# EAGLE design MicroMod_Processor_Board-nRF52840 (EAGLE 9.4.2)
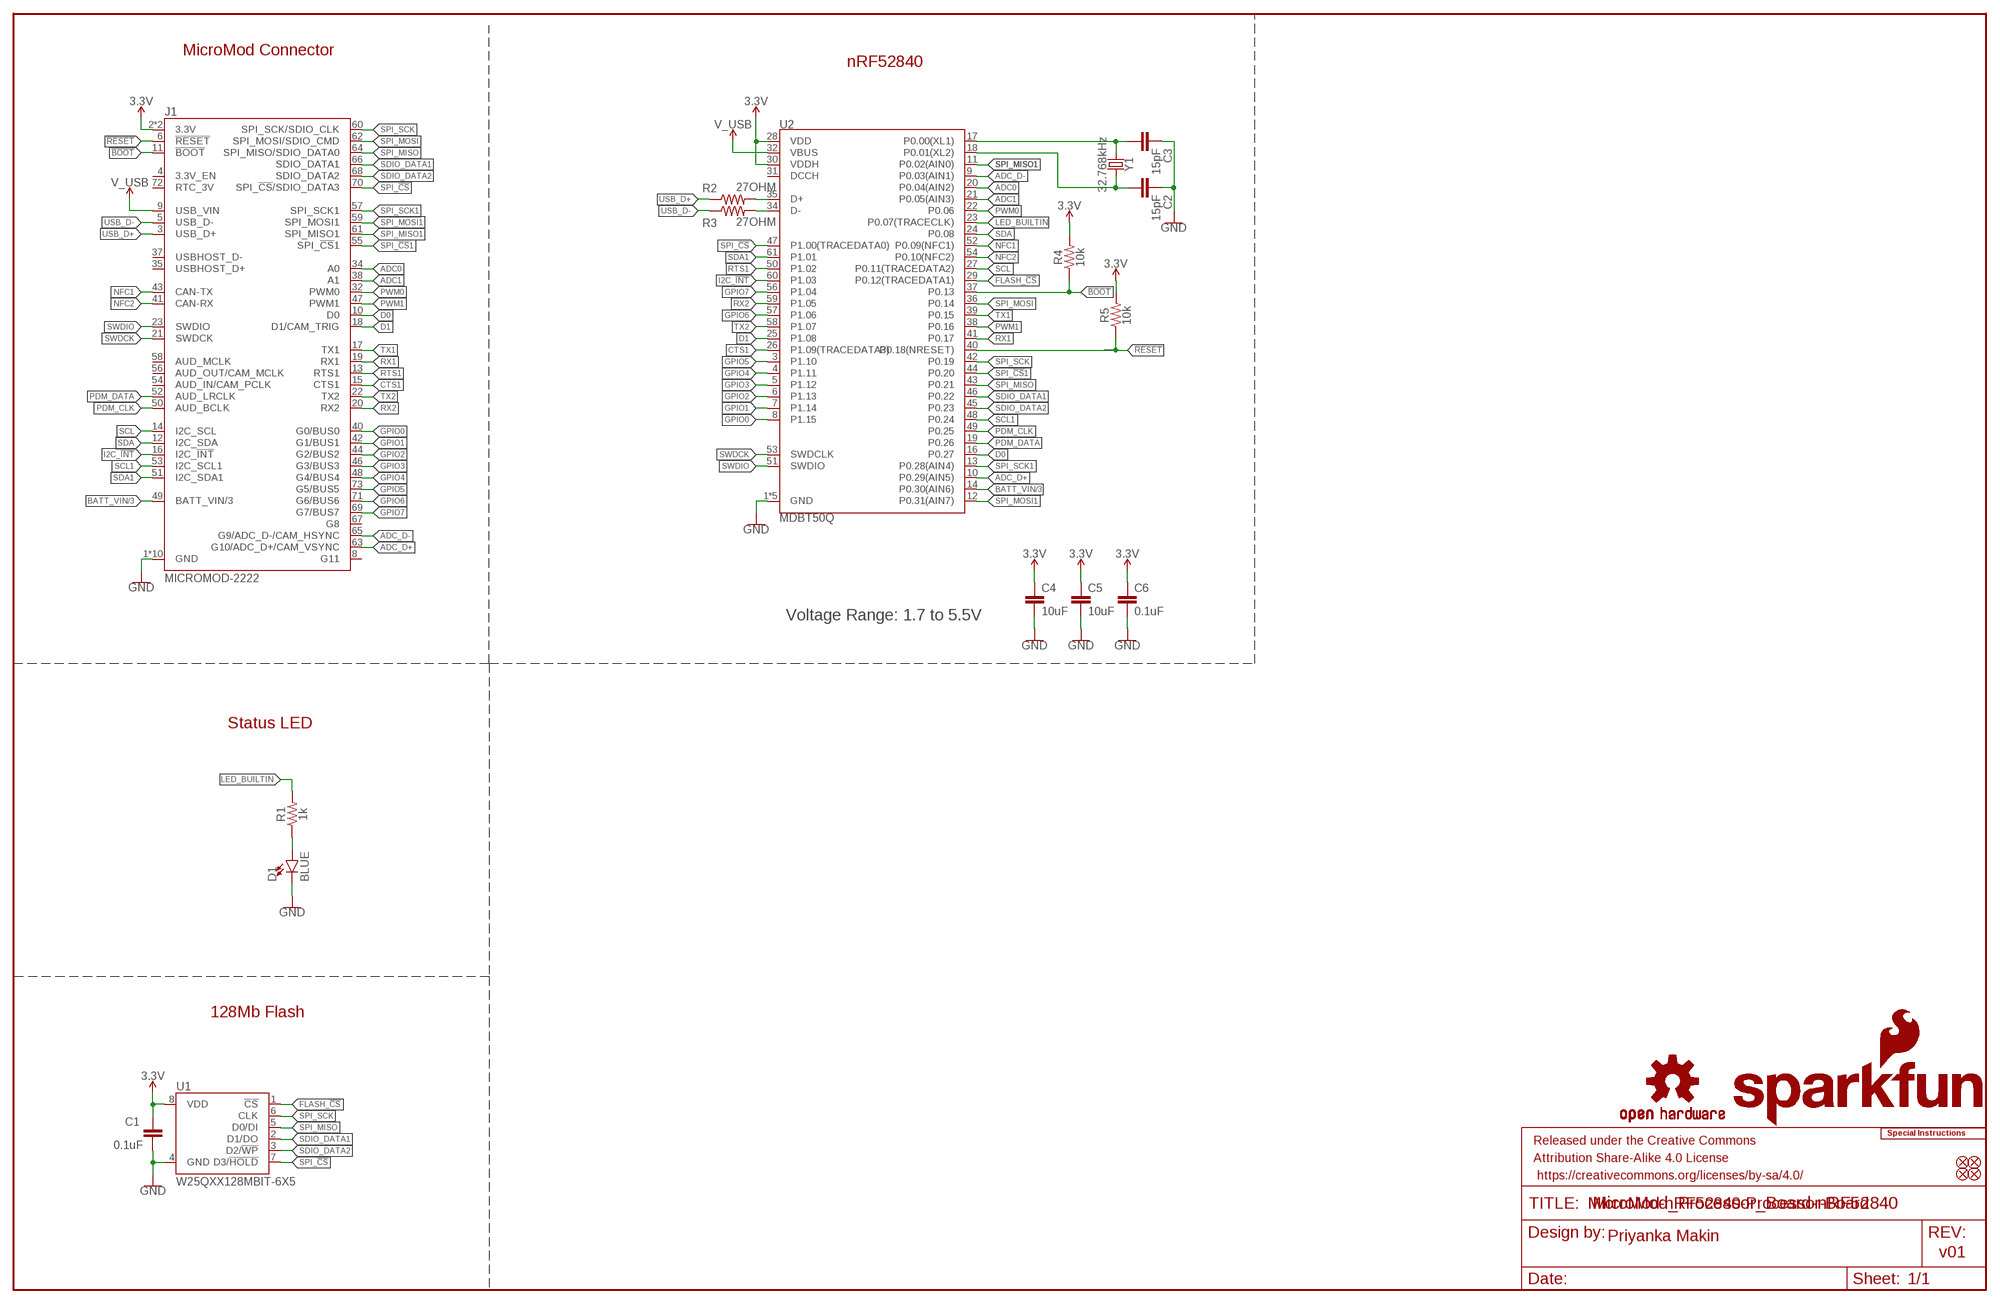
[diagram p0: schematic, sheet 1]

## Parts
C1  0.1uF  0.1UF-0402T-16V-10%  [0402-TIGHT]
C2  15pF  15PF-0402T-50V-5%  [0402-TIGHT]
C3  15pF  15PF-0402T-50V-5%  [0402-TIGHT]
C4  10uF  10UF-0402T-6.3V-20%  [0402-TIGHT]
C5  10uF  10UF-0402T-6.3V-20%  [0402-TIGHT]
C6  0.1uF  0.1UF-0402T-16V-10%  [0402-TIGHT]
D1  BLUE  LED-BLUE0603  [LED-0603]
FD1  FIDUCIALUFIDUCIAL  [FIDUCIAL-MICRO]
FD2  FIDUCIALUFIDUCIAL  [FIDUCIAL-MICRO]
FD3  FIDUCIALUFIDUCIAL  [FIDUCIAL-MICRO]
FD4  FIDUCIALUFIDUCIAL  [FIDUCIAL-MICRO]
FRAME1  FRAME-LEDGER  [CREATIVE_COMMONS]
J1  MICROMOD-2222  [M.2-CARD-E-22]
LOGO1  SFE_LOGO_NAME_FLAME.1_INCH  [SFE_LOGO_NAME_FLAME_.1]
LOGO2  SFE_LOGO_FLAME.1_INCH  [SFE_LOGO_FLAME_.1]
LOGO3  OSHW-LOGOMINI  [OSHW-LOGO-MINI]
LOGO4  SPECIAL_INSTRUCTIONS-ORDERING  [ORDERING_INSTRUCTIONS]
R1  1k  1KOHM-0402T-1/16W-1%  [0402-TIGHT]
R2  27OHM  [0402-TIGHT]
R3  27OHM  [0402-TIGHT]
R4  10k  10KOHM-0402T-1/16W-1%  [0402-TIGHT]
R5  10k  10KOHM-0402T-1/16W-1%  [0402-TIGHT]
U1  W25QXX128MBIT-6X5  [WSON-8-6X5]
U2  MDBT50Q  [MDBT50Q]
Y1  32.768kHz  CRYSTAL-32.768KHZSMD-3.2X1.5  [CRYSTAL-SMD-3.2X1.5MM]

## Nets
3.3V: C1.1 C4.1 C5.1 C6.1 J1.2(3.3V) J1.74(3.3V) R4.2 R5.2 U1.8(VDD) U2.28(VDD) U2.30(VDDH)
!BOOT!: J1.11(!BOOT!) R4.1 U2.37(P0.13)
!RESET!: J1.6(!RESET!) R5.1 U2.40(P0.18(NRESET))
ADC0: J1.34(A0) U2.20(P0.04(AIN2))
ADC1: J1.38(A1) U2.21(P0.05(AIN3))
ADC_D+: J1.63(G10/ADC_D+/CAM_VSYNC) U2.10(P0.29(AIN5))
ADC_D-: J1.65(G9/ADC_D-/CAM_HSYNC) U2.9(P0.03(AIN1))
BATT_VIN/3: J1.49(BATT_VIN/3) U2.14(P0.30(AIN6))
CTS1: J1.15(CTS1) U2.26(P1.09(TRACEDATA3))
D0: J1.10(D0) U2.16(P0.27)
D1: J1.18(D1/CAM_TRIG) U2.25(P1.08)
FLASH_!CS!: U1.1(!CS!) U2.29(P0.12(TRACEDATA1))
GND: C1.2 C2.1 C3.1 C4.2 C5.2 C6.2 D1.C J1.1(GND) J1.7(GND) J1.33(GND) J1.36(GND) J1.39(GND) J1.45(GND) J1.75(GND) J1.GND1(GND) J1.GND2(GND) J1.GND3(GND) U1.4(GND) U2.1(GND) U2.2(GND) U2.15(GND) U2.33(GND) U2.55(GND)
GPIO0: J1.40(G0/BUS0) U2.8(P1.15)
GPIO1: J1.42(G1/BUS1) U2.7(P1.14)
GPIO2: J1.44(G2/BUS2) U2.6(P1.13)
GPIO3: J1.46(G3/BUS3) U2.5(P1.12)
GPIO4: J1.48(G4/BUS4) U2.4(P1.11)
GPIO5: J1.73(G5/BUS5) U2.3(P1.10)
GPIO6: J1.71(G6/BUS6) U2.57(P1.06)
GPIO7: J1.69(G7/BUS7) U2.56(P1.04)
I2C_!INT!: J1.16(I2C_!INT!) U2.60(P1.03)
LED_BUILTIN: R1.2 U2.23(P0.07(TRACECLK))
N$1: R2.2 U2.35(D+)
N$2: D1.A R1.1
N$3: R3.2 U2.34(D-)
N$4: C3.2 U2.17(P0.00(XL1)) Y1.P$1
N$6: C2.2 U2.18(P0.01(XL2)) Y1.P$2
NFC1: J1.43(CAN-TX) U2.52(P0.09(NFC1))
NFC2: J1.41(CAN-RX) U2.54(P0.10(NFC2))
PDM_CLK: J1.50(AUD_BCLK) U2.49(P0.25)
PDM_DATA: J1.52(AUD_LRCLK) U2.19(P0.26)
PWM0: J1.32(PWM0) U2.22(P0.06)
PWM1: J1.47(PWM1) U2.38(P0.16)
RTS1: J1.13(RTS1) U2.50(P1.02)
RX1: J1.19(RX1) U2.41(P0.17)
RX2: J1.20(RX2) U2.59(P1.05)
SCL: J1.14(I2C_SCL) U2.27(P0.11(TRACEDATA2))
SCL1: J1.53(I2C_SCL1) U2.48(P0.24)
SDA: J1.12(I2C_SDA) U2.24(P0.08)
SDA1: J1.51(I2C_SDA1) U2.61(P1.01)
SDIO_DATA1: J1.66(SDIO_DATA1) U1.2(D1/DO) U2.46(P0.22)
SDIO_DATA2: J1.68(SDIO_DATA2) U1.3(D2/!WP!) U2.45(P0.23)
SPI_!CS!: J1.70(SPI_!CS!/SDIO_DATA3) U1.7(D3/!HOLD!) U2.47(P1.00(TRACEDATA0))
SPI_!CS!1: J1.55(SPI_!CS!1) U2.44(P0.20)
SPI_MISO: J1.64(SPI_MISO/SDIO_DATA0) U1.5(D0/DI) U2.43(P0.21)
SPI_MISO1: J1.61(SPI_MISO1) U2.11(P0.02(AIN0))
SPI_MOSI: J1.62(SPI_MOSI/SDIO_CMD) U2.36(P0.14)
SPI_MOSI1: J1.59(SPI_MOSI1) U2.12(P0.31(AIN7))
SPI_SCK: J1.60(SPI_SCK/SDIO_CLK) U1.6(CLK) U2.42(P0.19)
SPI_SCK1: J1.57(SPI_SCK1) U2.13(P0.28(AIN4))
SWDCK: J1.21(SWDCK) U2.53(SWDCLK)
SWDIO: J1.23(SWDIO) U2.51(SWDIO)
TX1: J1.17(TX1) U2.39(P0.15)
TX2: J1.22(TX2) U2.58(P1.07)
USB_D+: J1.3(USB_D+) R2.1
USB_D-: J1.5(USB_D-) R3.1
V_USB: J1.9(USB_VIN) U2.32(VBUS)
Unconnected: J1.4(3.3V_EN) J1.8(G11) J1.35(USBHOST_D+) J1.37(USBHOST_D-) J1.54(AUD_IN/CAM_PCLK) J1.56(AUD_OUT/CAM_MCLK) J1.58(AUD_MCLK) J1.67(G8) J1.72(RTC_3V) U2.31(DCCH)

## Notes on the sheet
- MicroMod Connector
- nRF52840
- Voltage Range: 1.7 to 5.5V
- Status LED
- 128Mb Flash
- MicroMod-nRF52840-Processor-Board
- Priyanka Makin
- v01

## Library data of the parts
C1 C6 = SparkFun-Capacitors:0.1UF: 0.1µF ceramic capacitors; PROD_ID: CAP-12416
C2 C3 = SparkFun-Capacitors:15PF: 15pF ceramic capacitors; PROD_ID: CAP-13063
C4 C5 = SparkFun-Capacitors:10UF: 10.0µF ceramic capacitors; PROD_ID: CAP-14848
D1 = SparkFun-LED:LED-BLUE: Blue SMD LED; PROD_ID: DIO-08575
FD1-FD4 = SparkFun-Aesthetics:FIDUCIAL: Fiducial Alignment Points
FRAME1 = SparkFun-Aesthetics:FRAME-LEDGER: Schematic Frame - Ledger
J1 = SparkFun-MicroMod:MICROMOD: MicroMod Connector Description: A card edge connector and mating PCB connector to allow various MicroMod Processor Boards to be coupled with various carrier boards of different capabilities. Based on the M.2 standard.
LOGO1 = SparkFun-Aesthetics:SFE_LOGO_NAME_FLAME: SparkFun Font Logo w/ Flame
LOGO2 = SparkFun-Aesthetics:SFE_LOGO_FLAME: SparkFun Flame Logo
LOGO3 = SparkFun-Aesthetics:OSHW-LOGO: Open-Source Hardware (OSHW) Logo
LOGO4 = SparkFun-Aesthetics:SPECIAL_INSTRUCTIONS: Special Ordering/Production Instructions Alert
R1 = SparkFun-Resistors:1KOHM: 1kΩ resistor; PROD_ID: RES-14342
R2 R3 = SparkFun-Resistors:27OHM: 27Ω resistor
R4 R5 = SparkFun-Resistors:10KOHM: 10kΩ resistor; PROD_ID: RES-14241
U1 = SparkFun-MicroMod:W25QXX; PROD_ID: IC-15107
U2 = SparkFun-RF:MDBT50Q; PROD_ID: IC-14109
Y1 = SparkFun-Clocks:CRYSTAL-32.768KHZ: 32.768kHz Crystal; PROD_ID: XTAL-13062

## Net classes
0 default: width 0 mm, drill 0 mm

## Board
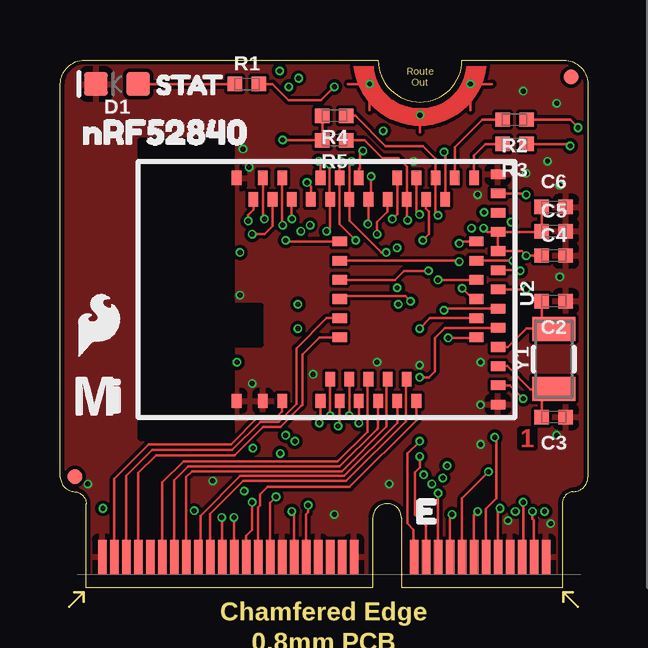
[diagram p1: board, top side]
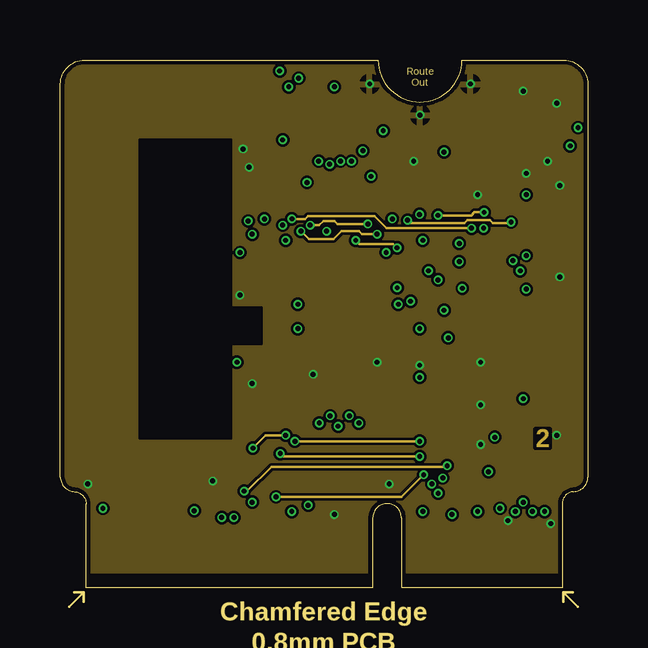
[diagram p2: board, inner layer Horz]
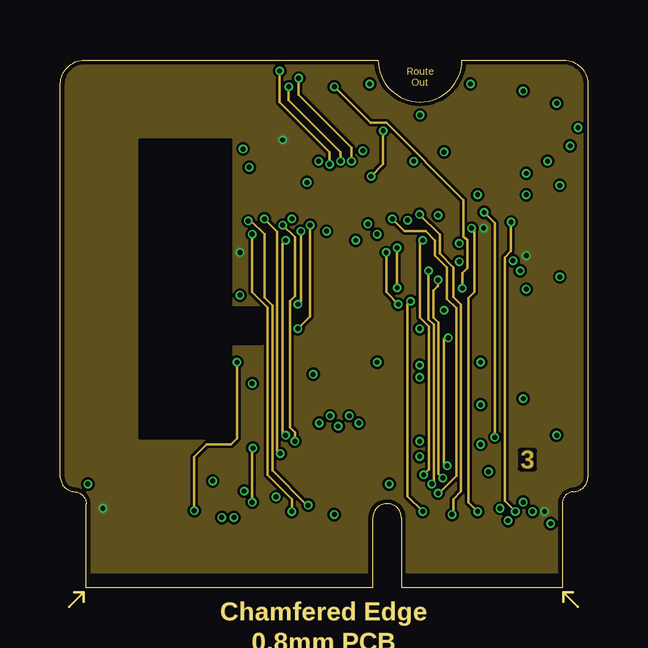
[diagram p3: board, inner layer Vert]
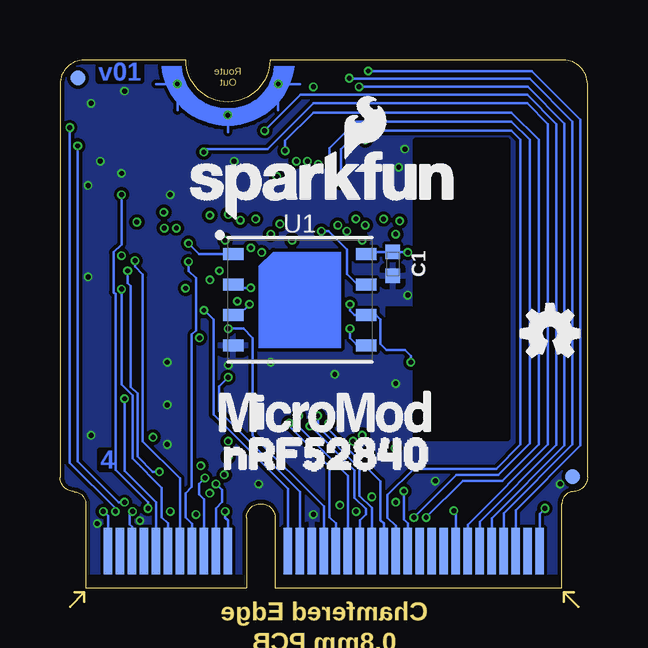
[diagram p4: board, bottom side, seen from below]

Size 22 x 22 mm. Coordinates in mm from the lower left corner, seen from the top.
Outline: 0,4.6 0,21 arc-87 1,22 13.25,22 arc180 16.75,22 21,22 arc-87 22,21 22,4.6
Outline: 0,4.6 arc87 0.6,4
Outline: 21.4,4 arc87 22,4.6
Outline: 21.4,4 arc85 20.93,3.5 20.93,0 14.22,0 14.22,2.9 arc180 13.03,2.9 13.03,0 1.07,0 1.07,3.5 arc84 0.6,4
Outline: 21.4,4 arc87 22,4.6
Outline: 0,4.6 arc87 0.6,4
Copper layers (1+2*15+16): Top 0.035mm / dielectric 1.5mm / Horz 0.035mm / dielectric 0.15mm / Vert 0.035mm / dielectric 0.2mm / Bottom 0.035mm
Design rules "SparkFun-4-layer-MicroMod": minimum track width 4mil, minimum drill 0.2mm, track to track 4mil, track to pad 4mil, pad to pad 4mil, via to via 4mil, smd to smd 4mil, copper to edge 6mil, drill to drill 6mil, minimum pad ring 3mil, minimum via ring 3mil, stop-mask expansion 4mil, vias tented up to drill 25mil, thermal gap 10mil

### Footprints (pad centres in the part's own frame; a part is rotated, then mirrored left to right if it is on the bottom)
0402-TIGHT = smd 0.6 x 0.6: 1 -0.5,0; 2 0.5,0
LED-0603 = smd 1 x 1: A -0.877,0; C 0.877,0
FIDUCIAL-MICRO = smd 0.635 x 0.635: 1 0,0
M.2-CARD-E-22 = smd 0.35 x 1.45: 1 9.25,1.275; 3 8.75,1.275; 5 8.25,1.275; 7 7.75,1.275; 9 7.25,1.275; 11 6.75,1.275; 13 6.25,1.275; 15 5.75,1.275; 17 5.25,1.275; 19 4.75,1.275; 21 4.25,1.275; 23 3.75,1.275; 33 1.25,1.275; 35 0.75,1.275; 37 0.25,1.275; 39 -0.25,1.275; 41 -0.75,1.275; 43 -1.25,1.275; 45 -1.75,1.275; 47 -2.25,1.275; 49 -2.75,1.275; 51 -3.25,1.275; 53 -3.75,1.275; 55 -4.25,1.275; 57 -4.75,1.275; 59 -5.25,1.275; 61 -5.75,1.275; 63 -6.25,1.275; 65 -6.75,1.275; 67 -7.25,1.275; 69 -7.75,1.275; 71 -8.25,1.275; 73 -8.75,1.275; 75 -9.25,1.275 | smd 0.35 x 1.95 bottom: 2 9,1.525; 4 8.5,1.525; 6 8,1.525; 8 7.5,1.525; 10 7,1.525; 12 6.5,1.525; 14 6,1.525; 16 5.5,1.525; 18 5,1.525; 20 4.5,1.525; 22 4,1.525; 32 1.5,1.525; 34 1,1.525; 36 0.5,1.525; 38 0,1.525; 40 -0.5,1.525; 42 -1,1.525; 44 -1.5,1.525; 46 -2,1.525; 48 -2.5,1.525; 50 -3,1.525; 52 -3.5,1.525; 54 -4,1.525; 56 -4.5,1.525; 58 -5,1.525; 60 -5.5,1.525; 62 -6,1.525; 64 -6.5,1.525; 66 -7,1.525; 68 -7.5,1.525; 70 -8,1.525; 72 -8.5,1.525; 74 -9,1.525 | drill 0.2: GND1 1.9,21; GND2 4,19.7; GND3 6.1,21
WSON-8-6X5 = smd 0.85 x 0.5: 1 -2.775,1.905; 2 -2.775,0.635; 3 -2.775,-0.635; 4 -2.775,-1.905; 5 2.775,-1.905; 6 2.775,-0.635; 7 2.775,0.635; 8 2.775,1.905
MDBT50Q = smd 0.6 x 0.4: 1 -4.65,3.65; 2 -4.65,2.55; 3 -4.65,1.75; 4 -4.65,0.15; 5 -3.75,-0.25; 6 -4.65,-0.65; 7 -3.75,-1.05; 8 -4.65,-1.45; 9 -3.75,-1.85; 10 -4.65,-2.25; 11 -3.75,-2.65; 12 -4.65,-3.05; 13 -3.75,-3.45; 14 -4.65,-3.85; 34 4.65,-6.25; 35 4.65,-5.45; 36 3.75,-5.05; 37 4.65,-4.65; 38 3.75,-4.25; 39 4.65,-3.85; 40 3.75,-3.45; 41 4.65,-3.05; 42 3.75,-2.65; 43 3.75,-1.85; 44 4.65,-1.45; 45 3.75,-1.05; 46 4.65,-0.65; 47 3.75,-0.25; 48 4.65,0.15; 49 3.75,0.55; 50 3.75,1.35; 51 4.65,1.75; 52 3.75,2.15; 53 4.65,2.55; 54 3.75,2.95; 55 4.65,3.65 | smd 0.4 x 0.6: 15 -4.8,-7.25; 16 -4,-7.25; 17 -3.2,-7.25; 18 -2.4,-7.25; 19 -2,-6.35; 20 -1.6,-7.25; 21 -1.2,-6.35; 22 -0.8,-7.25; 23 -0.4,-6.35; 24 0,-7.25; 25 0.4,-6.35; 26 0.8,-7.25; 27 1.2,-6.35; 28 1.6,-7.25; 29 2,-6.35; 30 2.4,-7.25; 31 3.2,-7.25; 32 4,-7.25; 33 4.8,-7.25; 56 -2,-0.65; 57 -1.2,-0.65; 58 -0.4,-0.65; 59 0.4,-0.65; 60 1.2,-0.65; 61 2,-0.65
CRYSTAL-SMD-3.2X1.5MM = smd 1 x 1.8: P$1 -1.25,0; P$2 1.25,0

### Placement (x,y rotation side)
C1  8.12,13.49 270 bottom
C2  20.57,11.94 180 top
C3  20.57,7.11 180 top
C4  20.57,13.84 0 top
C5  20.57,14.86 0 top
C6  20.57,15.88 0 top
D1  2.37,21 180 top
FD1  0.62,4.62 0 top
FD2  21.3,21.3 0 top
FD3  21.25,21.25 0 bottom
FD4  0.62,4.62 0 bottom
FRAME1  not placed on the board
J1  11,0 0 top
LOGO1  11,16.79 0 bottom
LOGO2  1.6,10.95 0 top
LOGO3  1.56,10.61 0 bottom
LOGO4  not placed on the board
R1  7.78,21 0 top
R2  18.94,19.51 180 top
R3  18.94,18.49 180 top
R4  11.43,19.67 180 top
R5  11.43,18.65 180 top
U1  12,12 0 bottom
U2  11,12.43 90 top
U$1  [MICROMOD_MI_LOGO_.35]  1.55,8 0 top
U$2  [NRF528400]  16.36,5.58 0 bottom
U$3  [NRF528400]  0,19 0 top
U$4  [STAT_TO_32]  3.25,20.96 0 top
U$5  [MICROMOD_LOGO_.35]  11,7.3 0 bottom
Y1  20.57,9.53 90 top

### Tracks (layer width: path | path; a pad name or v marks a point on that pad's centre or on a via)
3.3V  (via drill 0.2)
  Top 0.102: U2.30 20.05,14.83 C5.1 C6.1 | C4.1 v19.43,13.84 19.24,14.03 U2.28 U2.30 | R4.2 R5.2 9.29,18.65 v9.27,18.67 | U2.30 17.81,14.83 v17.65,14.99
  Bottom 0.102: J1.2 20,2.98 v20.19,3.17 | J1.74 2,3.08 v1.78,3.3 | U1.8 9.14,13.99 C1.1 7.52,13.99 v7.49,13.97
  pour Vert (isolate 0.102): 0,22 22,22 22,0.64 0,0.64
  cutout Vert (isolate 0.305): 3.3,18.67 7.11,18.67 7.11,11.68 8.38,11.68 8.38,10.16 7.11,10.16 7.11,6.22 3.3,6.22
!BOOT!  (via drill 0.2)
  Top 0.102: R4.1 12.31,19.67 13.56,18.41 15.11,18.41 15.65,17.88 U2.37 15.65,15.62 v15.75,15.52 | v18.12,6.27 18.19,6.2 18.19,3.71 17.75,3.27 J1.11
  Horz 0.102: v15.75,15.52 17.14,15.52 17.27,15.65 v17.67,15.65
  Vert 0.102: v17.67,15.65 18.12,15.2 v18.12,6.27
!RESET!  (via drill 0.2)
  Top 0.102: R5.1 12.69,18.65 13.44,17.91 14.1,17.91 14.45,17.55 U2.40 14.45,15.34 v14.48,15.32
  Horz 0.102: v18.8,15.24 18.75,15.19 18.03,15.19 17.91,15.32 16.97,15.32 16.84,15.19 14.61,15.19 v14.48,15.32
  Vert 0.102: v18.8,15.24 18.8,14.02 18.54,13.77 18.54,3.61 v18.97,3.17
  Bottom 0.102: v18.97,3.17 19.1,3.05 19.1,2.64 19,2.54 J1.6
ADC0  (via drill 0.2)
  Top 0.102: U2.20 16.04,10.83 15.62,10.41 15.62,9.02 15.37,8.76 v14.99,8.76
  Bottom 0.102: v14.99,8.76 15.37,8.38 15.37,7.37 12,4 J1.34
ADC1  (via drill 0.2)
  Top 0.102: U2.21 15.42,11.23 v14.99,10.79
  Bottom 0.102: v14.99,10.79 14.35,10.79 13.97,10.41 13.97,6.35 11,3.38 J1.38
ADC_D+
  Top 0.102: J1.63 4.75,4.47 5.33,5.05 11.65,5.05 13.2,6.6 13.21,6.6 13.25,6.65 U2.10
ADC_D-
  Top 0.102: J1.65 4.25,4.38 5.13,5.26 11.57,5.26 12.8,6.49 12.8,8.63 U2.9
BATT_VIN/3
  Top 0.102: U2.14 14.85,6.98 12.06,4.19 8.64,4.19 8.33,3.89 8.33,3.42 8.25,3.34 J1.49
CTS1  (via drill 0.2)
  Top 0.102: U2.26 19.16,13.23 v19.18,13.21 | J1.15 16.75,3.72 v17.86,4.83
  Bottom 0.102: v19.18,13.21 19.18,12.7 19.05,12.57 19.05,8.37 18.77,8.1 18.77,5.47 18.13,4.83 v17.86,4.83
D0  (via drill 0.2)
  Top 0.102: U2.16 18.75,8.43 v19.3,7.87
  Bottom 0.102: v19.3,7.87 19.3,4.86 18,3.56 J1.10
D1  (via drill 0.2)
  Top 0.102: U2.25 v15.75,12.83
  Vert 0.102: v15.95,4.57 15.77,4.75 15.77,11.05 15.56,11.27 15.56,12.38 15.75,12.57 v15.75,12.83
  Bottom 0.102: v15.95,4.57 16.2,4.32 16.2,3.89 16,3.68 J1.18
FLASH_!CS!  (via drill 0.2)
  Top 0.102: v16.64,14.35 16.72,14.43 U2.29
  Bottom 0.102: U1.1 16.19,13.9 v16.64,14.35
GND  (via drill 0.2)
  other vias: 7.62,18.29 13.21,9.4 14.99,9.27 11.43,3.05 20.45,2.67 18.67,2.79 7.49,12.19 20.83,16.76 20.83,12.95 19.43,17.27 17.53,7.62 8,8.51 7.87,17.53 14.73,17.78 19.3,20.7 20.7,20.19 20.32,17.78 17.4,16.38 1.14,4.32 6.35,4.45 13.72,4.32 10.54,8.89 17.53,5.97 17.53,9.4 20.7,6.35
  pour Top (isolate 0.14): 0,22 22,22 22,0.6 0,0.6
  pour Bottom (isolate 0.14): 0,22 22,22 22,0.6 0,0.6
  pour Horz (isolate 0.102): 0,0.64 0,22 22,22 22,0.64
  cutout Top (isolate 0.305): 3.3,18.67 7.11,18.67 7.11,11.68 8.38,11.68 8.38,10.16 7.11,10.16 7.11,6.22 3.3,6.22
  cutout Top (isolate 0.305): 3.3,18.67 7.11,18.67 7.11,11.68 8.38,11.68 8.38,10.16 7.11,10.16 7.11,6.22 3.3,6.22
  cutout Horz (isolate 0.305): 3.3,18.67 7.11,18.67 7.11,11.68 8.38,11.68 8.38,10.16 7.11,10.16 7.11,6.22 3.3,6.22
  cutout Bottom (isolate 0.305): 3.3,18.67 7.11,18.67 7.11,11.68 8.38,11.68 8.38,10.16 7.11,10.16 7.11,6.22 3.3,6.22
GPIO0  (via drill 0.2)
  Top 0.102: U2.8 v12.45,6.86
  Bottom 0.102: v12.45,6.86 12.45,6.73 10.75,5.04 10.75,2.92 10.5,2.67 J1.40
GPIO1  (via drill 0.2)
  Top 0.102: U2.7 v12.05,7.16
  Bottom 0.102: v12.05,7.16 12.05,6.72 10,4.67 J1.42
GPIO2  (via drill 0.2)
  Top 0.102: U2.6 11.65,6.8 v11.58,6.73
  Bottom 0.102: J1.44 9.5,2.79 9.25,3.05 9.25,3.28 9.71,3.74 9.71,4.89 11.55,6.73 v11.58,6.73
GPIO3  (via drill 0.2)
  Top 0.102: U2.5 v11.25,7.16
  Bottom 0.102: v11.25,7.16 11.25,6.72 9.5,4.97 9.51,4.97 9.51,3.83 9,3.32 J1.46
GPIO4  (via drill 0.2)
  Top 0.102: U2.4 10.85,6.91 v10.79,6.86
  Bottom 0.102: J1.48 8.5,2.67 8.63,2.79 8.63,4.44 10.79,6.6 v10.79,6.86
GPIO5
  Top 0.102: J1.73 2.25,4.54 3.68,5.97 7.11,5.97 8.26,7.11 9.02,7.11 9.25,7.34 U2.3
GPIO6
  Top 0.102: J1.71 2.75,4.66 3.83,5.74 7.17,5.74 8.34,6.91 9.1,6.91 9.84,7.65 9.84,9.97 11.1,11.23 U2.57
GPIO7
  Top 0.102: J1.69 3.25,4.77 3.99,5.51 7.26,5.51 8.45,6.71 9.19,6.71 10.05,7.57 10.1,7.62 10.1,9.72 10.81,10.43 U2.56
I2C_!INT!  (via drill 0.2)
  Top 0.102: U2.60 16.6,13.63 v16.64,13.59
  Bottom 0.102: v16.64,13.59 16.64,13.21 16.33,12.9 16.33,10.73 16.51,10.55 16.51,4.19 16.76,3.94 16.76,2.92 16.5,2.66 J1.16
LED_BUILTIN  (via drill 0.2)
  Top 0.102: R1.2 8.85,21 9.53,20.32 10.87,20.32 v11.43,20.88 | U2.23 17.21,12.03 v16.76,12.48
  Vert 0.102: v11.43,20.88 12.93,19.38 13.6,19.38 16.82,16.16 16.82,14.64 16.97,14.49 16.97,13.32 16.76,13.11 v16.76,12.48
N$1
  Top 0.102: R2.2 17.61,19.51 16.45,18.36 U2.35
N$2
  Top 0.102: D1.A R1.1
N$3
  Top 0.102: R3.2 17.73,18.49 17.25,18.01 U2.34
N$4
  Top 0.102: U2.17 18.63,9.23 19.61,8.26 20.55,8.26 Y1.P$1 20.07,7.78 C3.2
N$6
  Top 0.102: U2.18 18.67,10.03 19.43,10.79 20.55,10.79 Y1.P$2 20.07,11.28 C2.2
NFC1  (via drill 0.2)
  Top 0.102: U2.52 8.85,15.07 8.51,14.73 v8,14.73 | v9.65,3.17 9.75,3.08 J1.43
  Vert 0.102: v8,14.73 8,12.32 8.64,11.68 8.64,4.7 9.65,3.68 v9.65,3.17
NFC2  (via drill 0.2)
  Top 0.102: U2.54 8.05,15.76 7.83,15.54 v7.83,15.28 | v10.33,3.43 10.33,3.13 10.25,3.05 J1.41
  Vert 0.102: v7.83,15.28 7.96,15.28 8.51,14.73 8.51,12.1 8.84,11.77 8.84,4.88 10.29,3.43 v10.33,3.43
PDM_CLK  (via drill 0.2)
  Top 0.102: U2.49 10.45,16.73 v10.29,16.89
  Bottom 0.102: J1.50 8,2.57 8.34,2.9 8.34,3.85 7.24,4.95 3.81,4.95 2.79,5.97 2.79,18.67 3.17,19.05 9.53,19.05 10.29,18.29 v10.29,16.89
PDM_DATA  (via drill 0.2)
  Top 0.102: v16.18,10.41 17.33,10.41 U2.19
  Horz 0.102: v7.66,4.02 7.79,4.02 8.81,5.04 15.96,5.04 16,5.08 v16.13,5.08
  Vert 0.102: v16.13,5.08 16,5.21 16,10.36 16.05,10.41 v16.18,10.41
  Bottom 0.102: J1.52 7.5,2.67 7.66,2.84 v7.66,4.02
PWM0  (via drill 0.2)
  Top 0.102: v16,11.56 16.07,11.63 U2.22
  Bottom 0.102: J1.32 12.5,4.12 15.6,7.21 15.6,11.19 15.97,11.56 v16,11.56
PWM1  (via drill 0.2)
  Top 0.102: U2.38 15.25,15.8 15.38,15.67 15.38,14.74 v15.11,14.48 | J1.47 8.75,3.54 v8.99,3.78
  Horz 0.102: v8.99,3.78 14.23,3.78 v15.15,4.7
  Vert 0.102: v15.15,4.7 15.37,4.92 15.37,10.88 14.99,11.26 14.99,14.35 v15.11,14.48
RTS1  (via drill 0.2)
  Top 0.102: J1.13 17.25,3.03 v17.4,3.17 | v9.66,15.37 9.65,15.38 U2.50
  Horz 0.102: v9.66,15.37 10.2,15.37 10.33,15.49 13.09,15.49 13.6,14.99 v17.14,14.99
  Vert 0.102: v17.14,14.99 17.27,14.86 17.27,12.32 17.02,12.06 17.02,3.56 v17.4,3.17
RX1  (via drill 0.2)
  Top 0.102: U2.41 14.05,15.57 v13.84,15.37 | v15.75,3.93 J1.19
  Vert 0.102: v13.84,15.37 14.35,14.86 15.24,14.86 15.62,14.48 15.62,13.84 16.13,13.34 16.13,12.03 16.51,11.65 16.51,4.66 15.78,3.93 v15.75,3.93
RX2  (via drill 0.2)
  Top 0.102: U2.59 13.96,12.83 14.34,13.21 v15.35,13.21
  Vert 0.102: v15.35,13.21 15.35,11.18 15.57,10.96 15.57,4.32 v15.49,4.32
  Bottom 0.102: v15.49,4.32 15.24,4.06 15.24,3.56 15.5,3.3 J1.20
SCL  (via drill 0.2)
  Top 0.102: v18.87,13.63 U2.27
  Bottom 0.102: J1.14 17,4.55 18.54,6.1 18.54,13.05 18.87,13.38 v18.87,13.63
SCL1  (via drill 0.2)
  Top 0.102: J1.53 v7.25,2.91 v7.24,2.92 | U2.48 10.85,17.7 v10.77,17.78
  Bottom 0.102: v7.24,2.92 5.46,4.7 3.72,4.7 2.41,6 2.41,18.67 3.17,19.43 9.65,19.43 10.77,18.31 v10.77,17.78
SDA  (via drill 0.2)
  Top 0.102: U2.24 19.41,12.43 v19.43,12.45
  Bottom 0.102: v19.43,12.45 19.43,8.47 18.97,8.01 18.97,5.38 17.75,4.17 17.75,2.92 17.5,2.67 J1.12
SDA1  (via drill 0.2)
  Top 0.102: U2.61 9.35,14.43 v9.4,14.48 | v8,3.56 8,2.41 7.75,2.16 J1.51
  Horz 0.102: v9.4,6.35 8.56,6.35 v8.03,5.81
  Vert 0.102: v9.4,14.48 9.27,14.35 9.27,6.48 v9.4,6.35 | v8.03,5.81 8,5.79 v8,3.56
SDIO_DATA1  (via drill 0.2)
  Top 0.102: v12.32,14.48 11.65,15.15 U2.46 11.65,17.75 v11.68,17.78
  Horz 0.102: v14.04,14.17 13.88,14.33 12.47,14.33 v12.32,14.48
  Vert 0.102: v14.05,12.5 14.05,14.03 14.04,14.04 v14.04,14.17 | v11.68,17.78 11.68,18.16 9.53,20.32 v9.53,20.88
  Bottom 0.102: U1.2 14.64,12.5 v14.05,12.5 | J1.66 4,2.89 0.96,5.93 0.96,19.35 2.5,20.88 v9.53,20.88
SDIO_DATA2  (via drill 0.2)
  Top 0.102: v13.59,13.97 13.39,13.97 12.05,15.31 U2.45 12.05,17.69 v12.14,17.78
  Vert 0.102: v13.59,13.97 13.59,12.32 v14.1,11.81 | v12.14,17.78 12.14,18.34 9.94,20.54 v9.94,21.24
  Bottom 0.102: U1.3 14.54,11.37 v14.1,11.81 | J1.68 3.5,3.1 0.64,5.97 0.64,19.43 2.41,21.21 9.91,21.21 v9.94,21.24
SPI_!CS!  (via drill 0.2)
  Top 0.102: v11.23,17.65 11.23,16.2 U2.47 11.25,15.01 v11.1,14.86
  Vert 0.102: v11.23,17.65 11.23,18.16 9.14,20.24 v9.14,21.54
  Bottom 0.102: U1.7 9.59,12.63 10.03,13.08 10.03,14.1 10.79,14.86 v11.1,14.86 | J1.70 3,3.22 0.3,5.92 0.3,19.52 2.33,21.54 v9.14,21.54
SPI_!CS!1  (via drill 0.2)
  Top 0.102: J1.55 6.75,2.9 v6.73,2.92 | v12.61,18.21 12.48,18.09 12.48,17.5 12.45,17.46 U2.44
  Bottom 0.102: v6.73,2.92 5.21,4.45 3.56,4.45 2.03,5.97 2.03,18.67 3.17,19.81 11.43,19.81 12.61,18.63 v12.61,18.21
SPI_MISO  (via drill 0.2)
  Top 0.102: v12.83,15.16 12.85,15.16 U2.43 12.95,16.28 v12.95,17.14
  Horz 0.102: v12.83,15.16 11.56,15.16 11.43,15.29 10.97,15.29 10.79,15.11 v10.41,15.11
  Vert 0.102: v9.91,10.79 10.41,11.3 v10.41,15.11 | v13.46,19.05 13.46,17.65 v12.95,17.14
  Bottom 0.102: U1.5 9.29,10.16 9.65,10.16 9.91,10.41 v9.91,10.79 | J1.64 4.5,2.74 1.29,5.94 1.29,19.33 2.52,20.55 11.96,20.55 v13.46,19.05
SPI_MISO1
  Top 0.102: J1.61 5.25,4.62 5.49,4.85 11.74,4.85 13.6,6.71 13.6,8.63 U2.11
SPI_MOSI  (via drill 0.2)
  Top 0.102: v16,18.16 16.05,18.11 U2.36
  Bottom 0.102: J1.62 5,2.62 1.65,5.97 1.65,19.33 2.52,20.19 11.43,20.19 13.34,18.29 15.88,18.29 v16,18.16
SPI_MOSI1
  Top 0.102: U2.12 14.05,6.87 11.83,4.65 7.49,4.65 5.84,3 5.84,1.37 J1.59
SPI_SCK  (via drill 0.2)
  Top 0.102: U2.42 13.65,15.68 13.21,15.24 v13.21,14.73
  Horz 0.102: v13.21,14.73 12.57,14.73 12.45,14.86 11.72,14.86 11.39,14.53 10.36,14.53 v10.03,14.86
  Vert 0.102: v10.03,14.86 10.03,11.94 v9.91,11.81 | v5.58,3.2 5.58,5.45 6.1,5.97 7.11,5.97 7.37,6.22 v7.37,9.4
  Bottom 0.102: v9.91,11.81 9.91,11.56 9.71,11.37 U1.6 8.82,11.37 8.64,11.18 8.64,10.16 8.38,9.91 7.62,9.91 7.37,9.65 v7.37,9.4 | J1.60 5.5,3.12 v5.58,3.2
SPI_SCK1
  Top 0.102: J1.57 6.25,3.08 7.62,4.45 11.91,4.45 14.4,6.94 14.4,8.63 U2.13
SWDCK  (via drill 0.2)
  Top 0.102: U2.53 8.45,15.43 v8.51,15.37 | v14.99,5.46 14.99,5 14.78,4.8 14.78,3.04 15.25,2.57 J1.21
  Horz 0.102: v14.99,5.46 9.3,5.46 v9.17,5.59
  Vert 0.102: v8.51,15.37 9.04,14.83 9.04,5.71 v9.17,5.59
SWDIO  (via drill 0.2)
  Top 0.102: J1.23 14.73,1.29 14.73,2.41 14.48,2.67 14.48,5.59 v14.99,6.1 | U2.51 9.25,15.13 v9.27,15.11
  Horz 0.102: v9.78,6.1 v14.99,6.1
  Vert 0.102: v9.27,15.11 9.78,14.61 9.78,12.15 9.58,11.95 9.58,6.68 9.78,6.48 v9.78,6.1
TX1  (via drill 0.2)
  Top 0.102: U2.39 14.85,15.69 v14.98,15.56 | v16.33,3.05 16.25,2.97 J1.17
  Vert 0.102: v14.98,15.56 15.82,14.71 15.82,13.93 16.4,13.35 16.4,12.12 16.71,11.81 16.71,4.01 16.38,3.68 16.38,3.1 v16.33,3.05
TX2  (via drill 0.2)
  Top 0.102: U2.58 11.78,12.16 14.39,12.16 v14.61,11.94
  Vert 0.102: v14.61,11.94 14.48,11.81 14.48,3.81 v15.11,3.17
  Bottom 0.102: J1.22 15,2.79 15.11,2.91 v15.11,3.17
USB_D+  (via drill 0.2)
  Top 0.102: v21.59,19.18 21.26,19.51 R2.1 | J1.3 19.75,2.8 19.68,2.86 v19.68,3.17
  Bottom 0.102: v21.59,19.18 21.59,5.21 19.68,3.3 v19.68,3.17
USB_D-  (via drill 0.2)
  Top 0.102: v21.26,18.41 21.18,18.49 R3.1 | v19.3,3.56 19.3,1.33 J1.5
  Bottom 0.102: v21.26,18.41 21.26,5.26 19.56,3.56 v19.3,3.56
V_USB  (via drill 0.2)
  Top 0.102: U2.32 19.38,16.43 v19.43,16.38 | J1.9 18.25,3.22 v18.33,3.3
  Bottom 0.102: v19.43,16.38 19.43,14.31 19.76,13.98 19.76,12.31 19.68,12.23 19.68,4.91 18.33,3.56 v18.33,3.3

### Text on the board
Top: 1
Horz: 2
Vert: 3
Bottom: v01 | 4
tDocu: 0.8mm PCB / 45 degree chamfered edge / Four layer design | Priyanka Makin

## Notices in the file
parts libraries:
SparkFun-Aesthetics: Licensing: Creative Commons ShareAlike 4.0 International - https://creativecommons.org/licenses/by-sa/4.0
SparkFun-Aesthetics: Released under the Creative Commons Attribution Share-Alike 4.0 License
SparkFun-Aesthetics: https://creativecommons.org/licenses/by-sa/4.0
